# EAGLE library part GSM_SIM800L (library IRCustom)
SIM800K Quad-Band GSM/GPRS Module 850/900/1800/1900 MHz Bluetooth EDR (3.0) FM Band: 76-109MHz (50kHz steps) -40 - 85°C
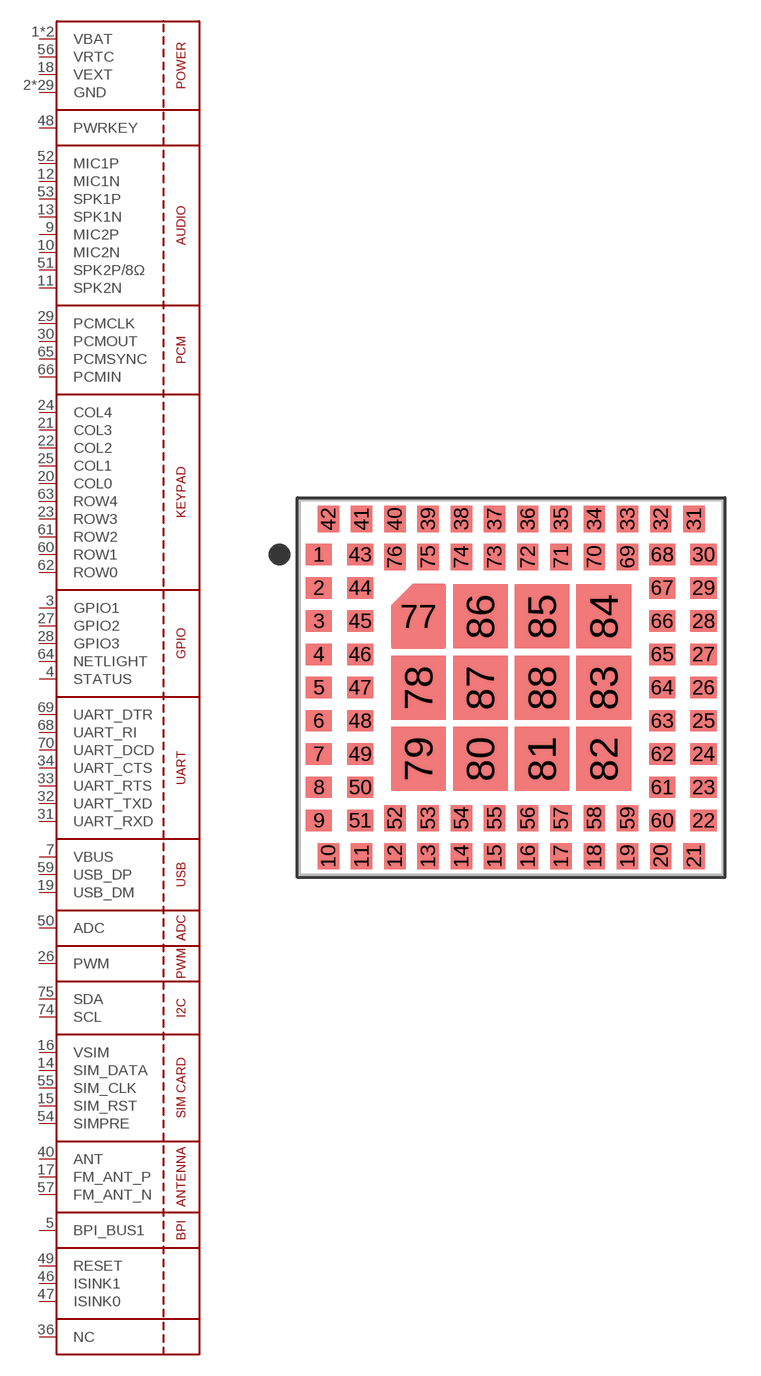
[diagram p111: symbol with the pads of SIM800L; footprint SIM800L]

Designator prefix U

## GSM_SIM800L  [SIM800L]
1  VBAT  pwr
2  GND  pwr
3  GPIO1
4  STATUS  out
5  BPI_BUS1  out
6  GND  pwr
7  VBUS  pwr
8  GND  pwr
9  MIC2P  in
10  MIC2N  in
11  SPK2N  out
12  MIC1N  in
13  SPK1N  out
14  SIM_DATA
15  SIM_RST  out
16  VSIM  pwr
17  FM_ANT_P
18  VEXT  pwr
19  USB_DM
20  COL0
21  COL3
22  COL2
23  ROW3
24  COL4
25  COL1
26  PWM  out
27  GPIO2
28  GPIO3
29  PCMCLK  out
30  PCMOUT  out
31  UART_RXD  in
32  UART_TXD  out
33  UART_RTS  in
34  UART_CTS  out
35  GND  pwr
36  NC  nc
37  GND  pwr
38  GND  pwr
39  GND  pwr
40  ANT
41  GND  pwr
42  VBAT  pwr
43  GND  pwr
44  GND  pwr
45  GND  pwr
46  ISINK1  in
47  ISINK0  in
48  PWRKEY  in
49  RESET  in
50  ADC  in
51  SPK2P/8Ω  out
52  MIC1P  in
53  SPK1P  out
54  SIMPRE  in
55  SIM_CLK  out
56  VRTC  pwr
57  FM_ANT_N
58  GND  pwr
59  USB_DP
60  ROW1
61  ROW2
62  ROW0
63  ROW4
64  NETLIGHT  out
65  PCMSYNC  out
66  PCMIN  in
67  GND  pwr
68  UART_RI  out
69  UART_DTR  in
70  UART_DCD  in
71  GND  pwr
72  GND  pwr
73  GND  pwr
74  SCL
75  SDA
76  GND  pwr
77  GND  pwr
78  GND  pwr
79  GND  pwr
80  GND  pwr
81  GND  pwr
82  GND  pwr
83  GND  pwr
84  GND  pwr
85  GND  pwr
86  GND  pwr
87  GND  pwr
88  GND  pwr

## Footprint SIM800L (pad centres in mm)
smd 1.1 x 0.9: 1 -8.1,5.6; 2 -8.1,4.2; 3 -8.1,2.8; 4 -8.1,1.4; 5 -8.1,0; 6 -8.1,-1.4; 7 -8.1,-2.8; 8 -8.1,-4.2; 9 -8.1,-5.6; 22 8.1,-5.6; 23 8.1,-4.2; 24 8.1,-2.8; 25 8.1,-1.4; 26 8.1,0; 27 8.1,1.4; 28 8.1,2.8; 29 8.1,4.2; 30 8.1,5.6; 43 -6.36,5.6; 44 -6.36,4.2; 45 -6.36,2.8; 46 -6.36,1.4; 47 -6.36,0; 48 -6.36,-1.4; 49 -6.36,-2.8; 50 -6.36,-4.2; 51 -6.36,-5.6; 60 6.36,-5.6; 61 6.36,-4.2; 62 6.36,-2.8; 63 6.36,-1.4; 64 6.36,0; 65 6.36,1.4; 66 6.36,2.8; 67 6.36,4.2; 68 6.36,5.6
smd 0.9 x 1.1: 10 -7.7,-7.1; 11 -6.3,-7.1; 12 -4.9,-7.1; 13 -3.5,-7.1; 14 -2.1,-7.1; 15 -0.7,-7.1; 16 0.7,-7.1; 17 2.1,-7.1; 18 3.5,-7.1; 19 4.9,-7.1; 20 6.3,-7.1; 21 7.7,-7.1; 31 7.7,7.1; 32 6.3,7.1; 33 4.9,7.1; 34 3.5,7.1; 35 2.1,7.1; 36 0.7,7.1; 37 -0.7,7.1; 38 -2.1,7.1; 39 -3.5,7.1; 40 -4.9,7.1; 41 -6.3,7.1; 42 -7.7,7.1; 52 -4.9,-5.5; 53 -3.5,-5.5; 54 -2.1,-5.5; 55 -0.7,-5.5; 56 0.7,-5.5; 57 2.1,-5.5; 58 3.5,-5.5; 59 4.9,-5.5; 69 4.9,5.5; 70 3.5,5.5; 71 2.1,5.5; 72 0.7,5.5; 73 -0.7,5.5; 74 -2.1,5.5; 75 -3.5,5.5; 76 -4.9,5.5
smd 1.5 x 1.5: 77 -3.9,3
smd 2.3 x 2.7: 78 -3.9,0; 79 -3.9,-3; 80 -1.3,-3; 81 1.3,-3; 82 3.9,-3; 83 3.9,0; 84 3.9,3; 85 1.3,3; 86 -1.3,3; 87 -1.3,0; 88 1.3,0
